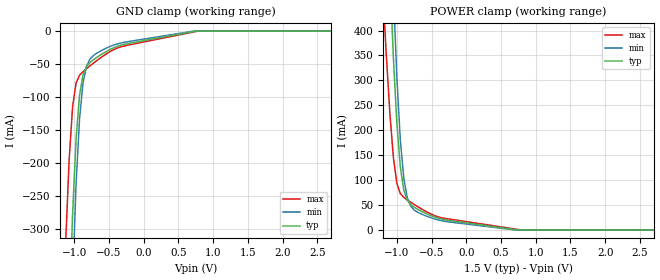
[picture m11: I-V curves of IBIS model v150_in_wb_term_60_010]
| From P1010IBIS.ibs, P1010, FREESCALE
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[Model]  v150_in_wb_term_60_010
|   Model v150_in_wb_term_60_010
| This model has derived from v150_wb_term_60_010
| Only applicable curves and parameters are copied
Model_type Input
Polarity   Non-Inverting
Enable   Active-High
Vinl =   0.5750V
Vinh =   0.9250V
C_comp   1.9143pF   1.6816pF   2.2180pF
[Receiver Thresholds]
Vth   =  0.750V
Vinh_ac  =  0.175V
Vinh_dc  =  0.100V
Vinl_ac  = -0.175V
Vinl_dc  = -0.100V
[Temperature Range]   65.0000   0.1050k   -40.0000
[Voltage Range]   1.5000V   1.4250V   1.5750V
[GND_clamp]
|Voltage   I(typ)   I(min)   I(max)
-1.575V   -3.171A    -3.724A    -2.089A
-1.125V   -637.9mA   -816.2mA   -320.9mA
-1.075V   -438.4mA   -579.2mA   -195.8mA
-1.025V   -277.5mA   -381.9mA   -114.5mA
-975mV    -163.5mA   -232.1mA   -78.83mA
-925mV    -97.28mA   -133.3mA   -67.11mA
-875mV    -66.58mA   -78.81mA   -61.63mA
-825mV    -53.85mA   -53.56mA   -57.14mA
-675mV    -39.78mA   -33.38mA   -44.64mA
-325mV    -21.28mA   -17.96mA   -23.75mA
775mV     0A         0A         -156.7uA
3.15V     0A         0A         0A
[POWER_clamp]
|Voltage   I(typ)   I(min)   I(max)
-1.575V   2.905A     3.676A     1.634A
-1.2V     933.8mA    1.225A     475.6mA
-1.15V    714mA      948.7mA    346.5mA
-1.1V     515.8mA    698.3mA    233.5mA
-1.05V    346.4mA    481.5mA    145.7mA
-1V       214.6mA    306.8mA    93.72mA
-950mV    126.8mA    181mA      73.06mA
-900mV    80mA       103.9mA    65.33mA
-800mV    50.66mA    47.74mA    55.65mA
-700mV    41.54mA    35.56mA    46.82mA
800mV     0A         0A         0A
3.15V     0A         0A         0A
